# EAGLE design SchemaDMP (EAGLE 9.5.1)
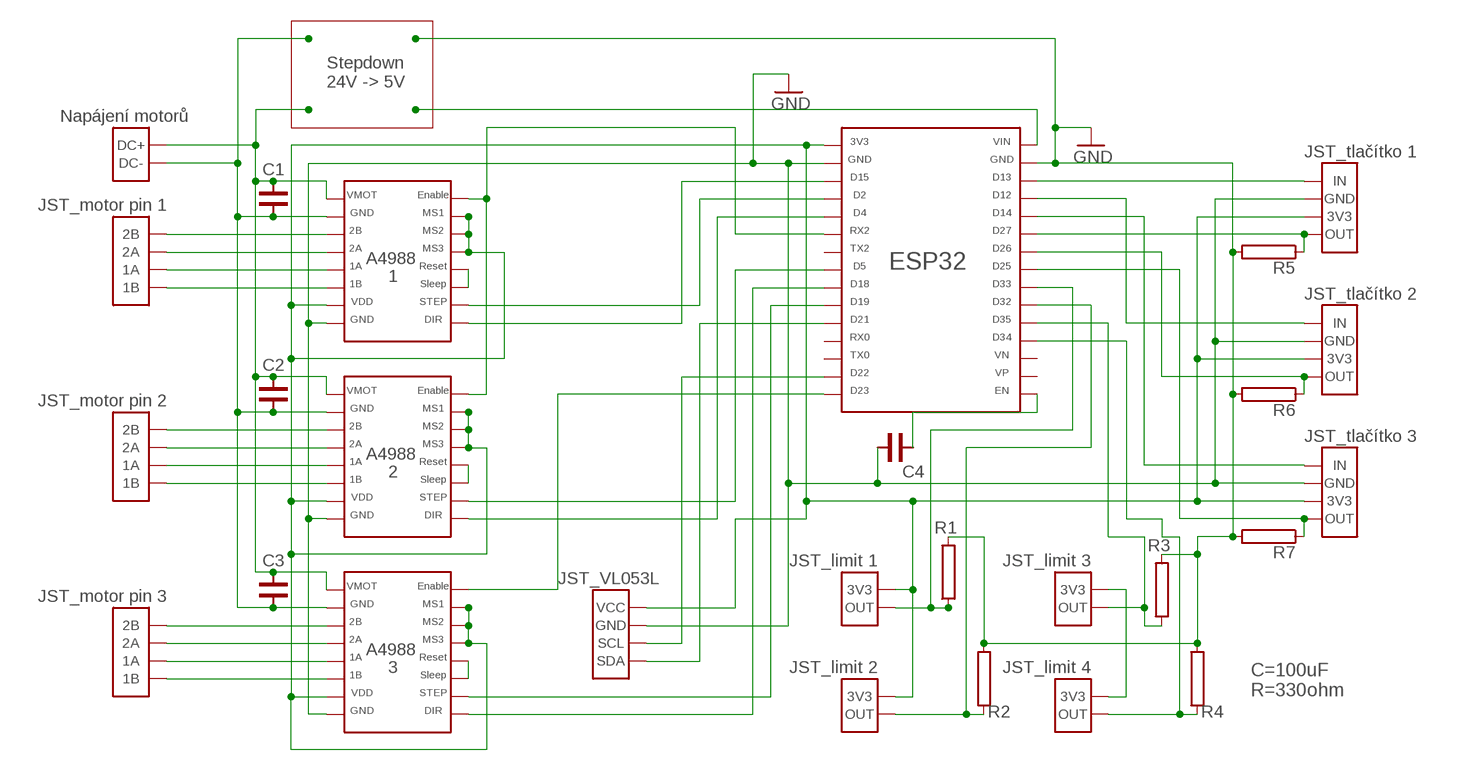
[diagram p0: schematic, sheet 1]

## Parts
R1  RR  [R]
R2  RR  [R]
R3  RR  [R]
R4  RR  [R]
R5  RR  [R]
R6  RR  [R]
R7  RR  [R]
U$1  A4988  [A4988]
U$2  A4988  [A4988]
U$3  JST_4P  [JST_4P]
U$4  JST_4P  [JST_4P]
U$5  A4988  [A4988]
U$6  JST_4P  [JST_4P]
U$7  POWER_2P  [POWER_2P]
U$8  ESP32  [ESP32]
U$9  JST_2P  [JST_2P]
U$10  JST_2P  [JST_2P]
U$11  JST_2P  [JST_2P]
U$12  JST_MOTOR  [JST_MOTOR]
U$13  JST_MOTOR  [JST_MOTOR]
U$14  JST_VL053L  [JST_VL053L]
U$15  JST_2P  [JST_2P]
U$16  JST_MOTOR  [JST_MOTOR]
U$18  C  [C]
U$19  C  [C]
U$20  C  [C]
U$22  STEPDOWN  [STEPDOWN]
U$23  C  [C]

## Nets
GND: R1.2 R2.2 R3.2 R4.2 R5.2 R6.2 R7.2 U$1.P$8(GND2) U$2.P$8(GND2) U$3.P$2 U$4.P$2 U$5.P$8(GND2) U$6.P$2 U$8.P$2(GND) U$8.P$17(GND2) U$14.P$2 U$22.P$1 U$23.P$1
N$2: U$1.P$2(GND) U$2.P$2(GND) U$5.P$2(GND) U$7.P$2 U$18.P$1 U$19.P$1 U$20.P$1 U$22.P$4
N$3: U$5.P$3(2B) U$12.P$1
N$4: U$5.P$4(2A) U$12.P$2
N$5: U$5.P$5(1A) U$12.P$3
N$6: U$5.P$6(1B) U$12.P$4
N$7: U$1.P$3(2B) U$13.P$1
N$8: U$1.P$4(2A) U$13.P$2
N$9: U$1.P$5(1A) U$13.P$3
N$10: U$1.P$6(1B) U$13.P$4
N$11: U$2.P$3(2B) U$16.P$1
N$12: U$2.P$4(2A) U$16.P$2
N$13: U$2.P$5(1A) U$16.P$3
N$14: U$2.P$6(1B) U$16.P$4
N$15: U$5.P$16(DIR) U$8.P$18(D15)
N$17: U$1.P$9(ENABLE) U$5.P$9(ENABLE) U$8.P$21(RX2)
N$19: U$1.P$7(VDD) U$1.P$10(MS1) U$1.P$11(MS2) U$1.P$12(MS3) U$2.P$7(VDD) U$2.P$10(MS1) U$2.P$11(MS2) U$2.P$12(MS3) U$3.P$3 U$4.P$3 U$5.P$7(VDD) U$5.P$10(MS1) U$5.P$11(MS2) U$5.P$12(MS3) U$6.P$3 U$8.P$16(3V3) U$10.P$1 U$14.P$1 U$15.P$1
N$21: U$5.P$13(RESET) U$5.P$14(SLEEP)
N$22: U$1.P$13(RESET) U$1.P$14(SLEEP)
N$23: U$2.P$13(RESET) U$2.P$14(SLEEP)
N$24: R5.1 U$4.P$4 U$8.P$6(D27)
N$25: U$5.P$15(STEP) U$8.P$19(D2)
N$26: U$1.P$16(DIR) U$8.P$20(D4)
N$27: U$1.P$15(STEP) U$8.P$23(D5)
N$28: U$2.P$15(STEP) U$8.P$25(D19)
N$29: U$2.P$16(DIR) U$8.P$24(D18)
N$30: U$8.P$1(VIN) U$22.P$2
N$31: R2.1 U$8.P$10(D32) U$10.P$2
N$32: R3.1 U$8.P$11(D35) U$9.P$2
N$33: R4.1 U$8.P$12(D34) U$11.P$2
N$34: U$8.P$26(D21) U$14.P$4
N$35: U$8.P$29(D22) U$14.P$3
N$36: U$4.P$1 U$8.P$3(D13)
N$37: U$6.P$1 U$8.P$4(D12)
N$38: U$3.P$1 U$8.P$5(D14)
N$39: R6.1 U$6.P$4 U$8.P$7(D26)
N$40: R7.1 U$3.P$4 U$8.P$8(D25)
N$41: U$2.P$9(ENABLE) U$8.P$30(D23)
N$44: U$8.P$15(EN) U$23.P$2
N$45: R1.1 U$8.P$9(D33) U$15.P$2
N$49: U$9.P$1 U$11.P$1
N$51: U$1.P$1(VMOT) U$2.P$1(VMOT) U$5.P$1(VMOT) U$7.P$1 U$18.P$2 U$19.P$2 U$20.P$2 U$22.P$3
Unconnected: U$8.P$13(VN) U$8.P$14(VP) U$8.P$22(TX2) U$8.P$27(RX0) U$8.P$28(TX0)

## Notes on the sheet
- Stepdown 
  24V -> 5V
- Napájení motorů
- JST_tlačítko 1
- C1
- JST_motor pin 1
- 1
- JST_tlačítko 2
- C2
- JST_motor pin 2
- JST_tlačítko 3
- 2 | C4
- C3 | JST_limit 1 | JST_limit 3
- JST_motor pin 3
- 3 | JST_limit 2 | JST_limit 4
- C=100uF
  R=330ohm

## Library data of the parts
R1-R7 = _DMP:R
U$1 U$2 U$5 = _DMP:A4988
U$3 U$4 U$6 = _DMP:JST_4P
U$7 = _DMP:POWER_2P
U$8 = _DMP:ESP32
U$9-U$11 U$15 = _DMP:JST_2P
U$12 U$13 U$16 = _DMP:JST_MOTOR
U$14 = _DMP:JST_VL053L
U$18-U$20 U$23 = _DMP:C
U$22 = _DMP:STEPDOWN

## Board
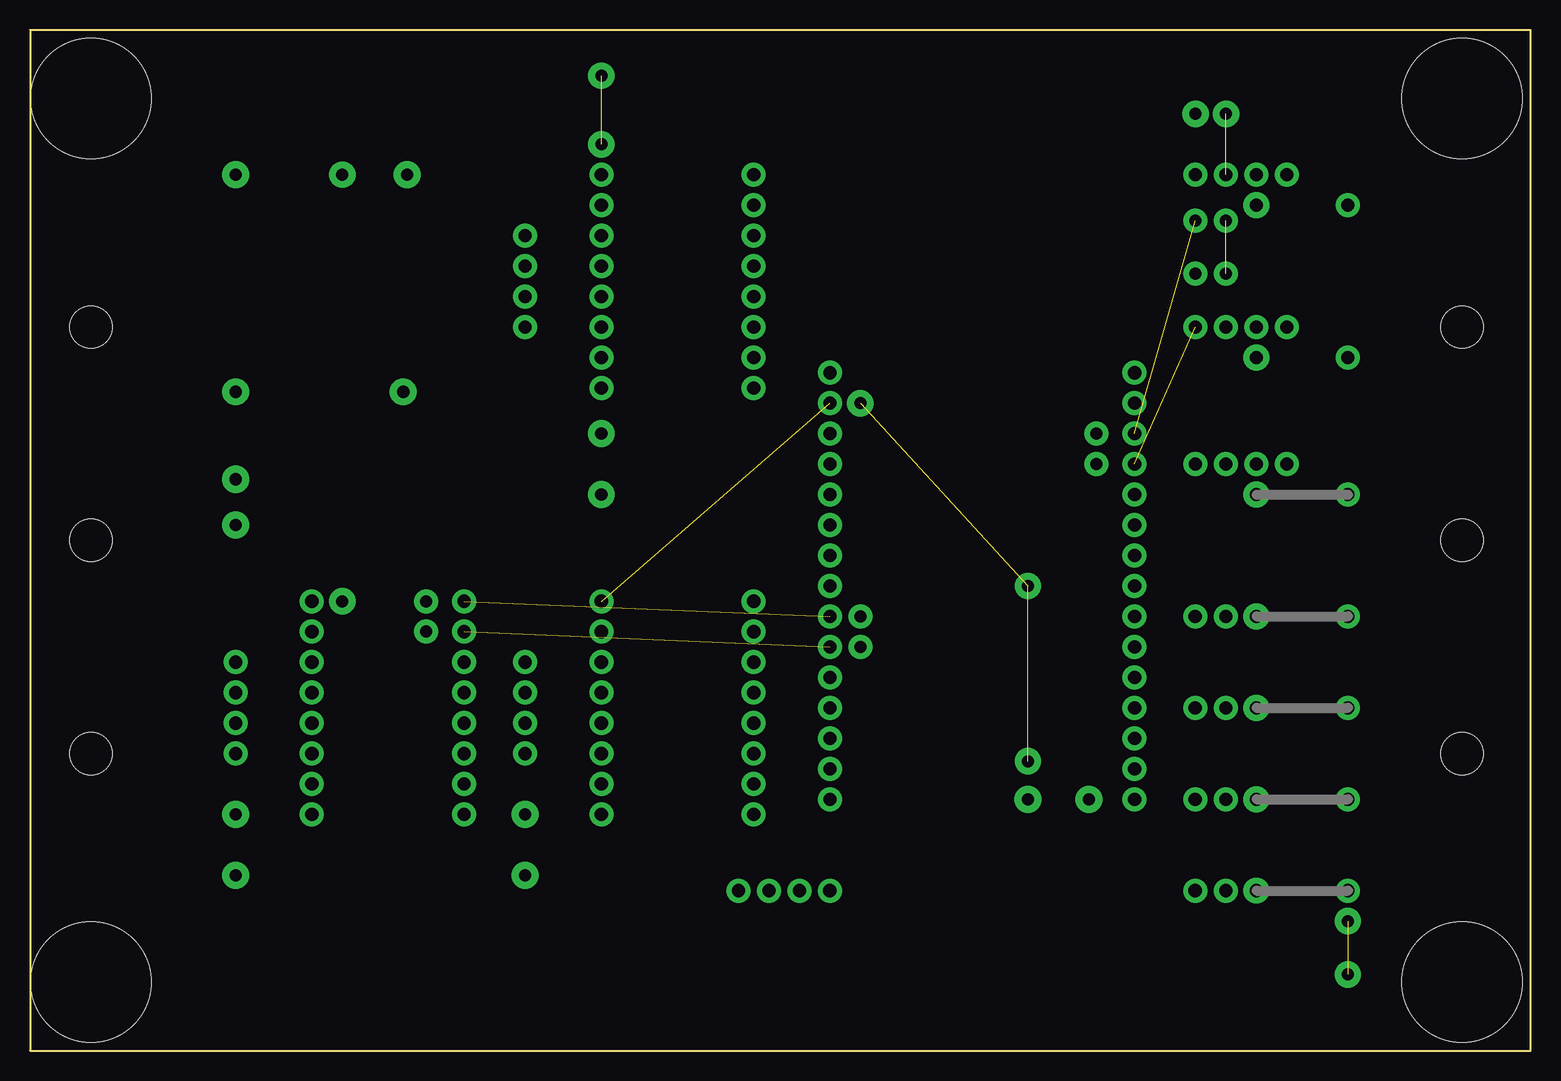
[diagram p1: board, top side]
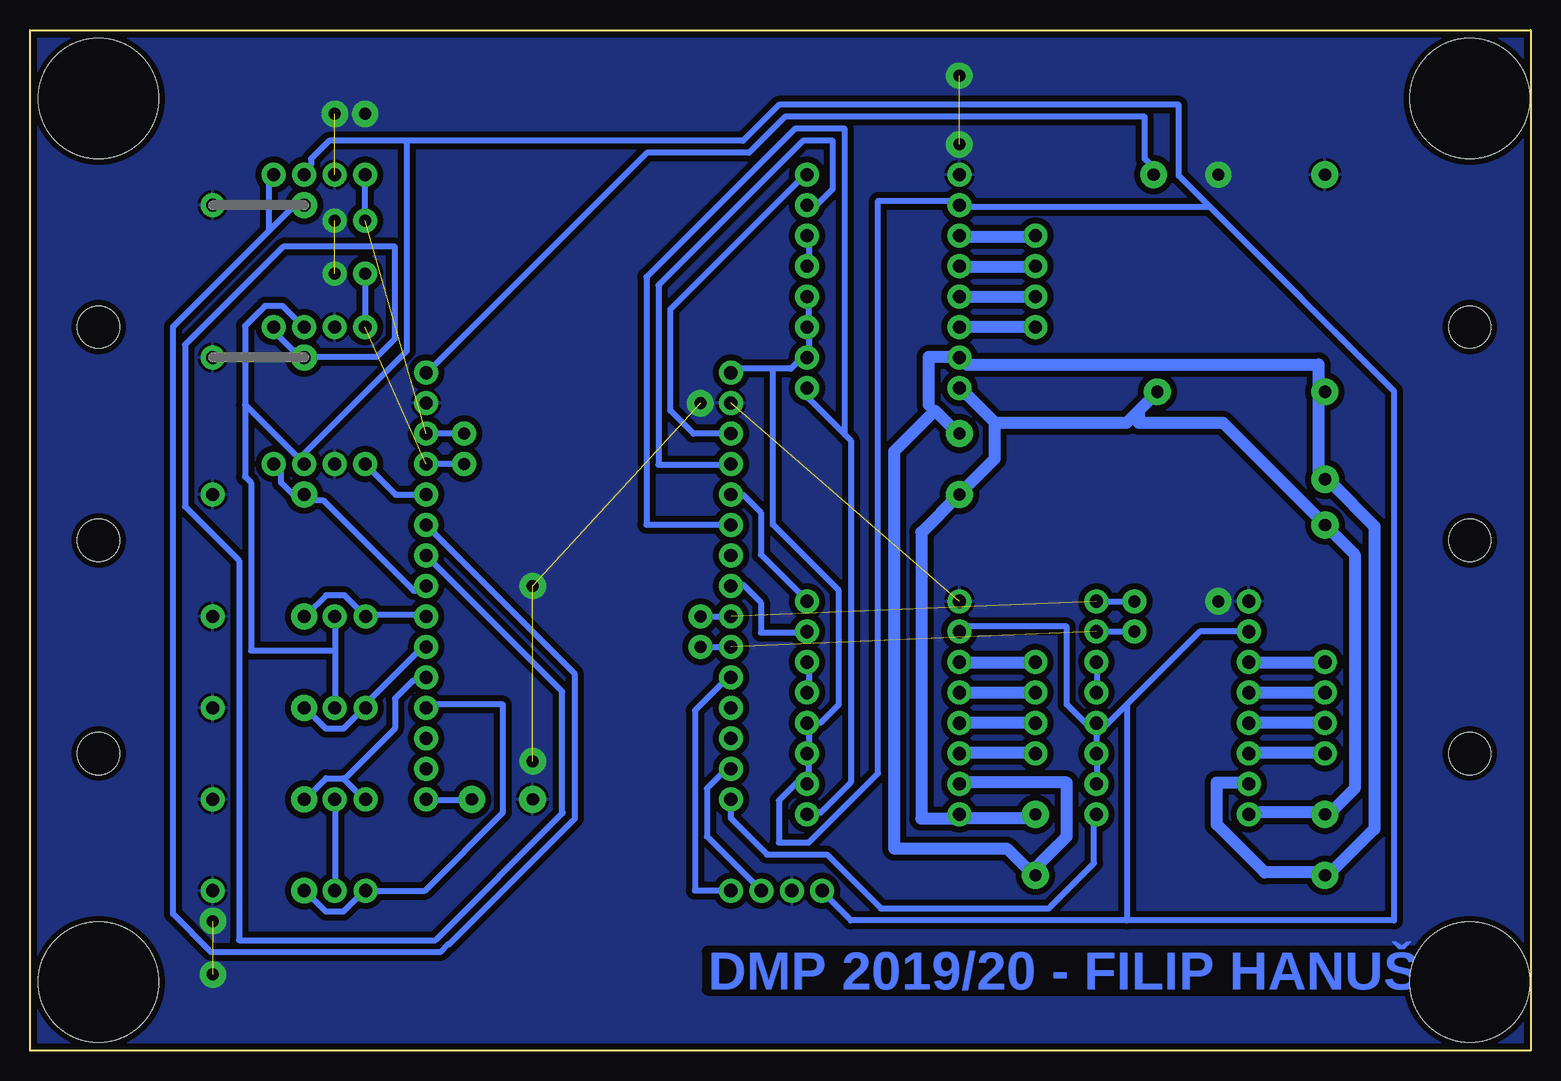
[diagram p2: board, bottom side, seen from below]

Size 125.09 x 85.09 mm. Coordinates in mm from the lower left corner, seen from the top.
Outline: 0,0 125.09,0 125.09,85.09 0,85.09 0,0
Copper layers (1*16): Top 0.035mm / dielectric 1.5mm / Bottom 0.035mm
Design rules "default *": minimum track width 0.5mm, minimum drill 1mm, track to track 0.5mm, track to pad 0.5mm, pad to pad 0.3mm, via to via 0.5mm, smd to smd 0.3mm, copper to edge 0.5mm, drill to drill 0.5mm, minimum pad ring 10mil, minimum via ring 8mil, stop-mask expansion 4mil, vias tented up to drill 0mil, thermal gap 10mil
Holes 3.5 mm at 5.08,42.55 119.38,42.55 5.08,60.33 5.08,24.77 119.38,60.33 119.38,24.77
Holes 10 mm at 5.08,79.38 119.38,79.38 119.38,5.71 5.08,5.71

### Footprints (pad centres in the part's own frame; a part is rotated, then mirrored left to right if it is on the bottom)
R = drill 1.1 pad 2.15: 1 0,0 | drill 1.1 pad 2: 2 7.62,0
A4988 = drill 1.1 pad 2: P$1 0,0; P$2 2.54,0; P$3 5.08,0; P$4 7.62,0; P$5 10.16,0; P$6 12.7,0; P$7 15.24,0; P$8 17.78,0; P$9 0,-12.7; P$10 2.54,-12.7; P$11 5.08,-12.7; P$12 7.62,-12.7; P$13 10.16,-12.7; P$14 12.7,-12.7; P$15 15.24,-12.7; P$16 17.78,-12.7
JST_4P = drill 1.1 pad 2: P$1 0,0; P$2 0,-2.54; P$3 0,-5.08; P$4 0,-7.62
POWER_2P = drill 1.02 pad 2.27: P$1 0,1.27; P$2 0,-2.54
ESP32 = drill 1.1 pad 2: P$1 0,0; P$2 2.54,0; P$3 5.08,0; P$4 7.62,0; P$5 10.16,0; P$6 12.7,0; P$7 15.24,0; P$8 17.78,0; P$9 20.32,0; P$10 22.86,0; P$11 25.4,0; P$12 27.94,0; P$13 30.48,0; P$14 33.02,0; P$15 35.56,0; P$16 0,-25.4; P$17 2.54,-25.4; P$18 5.08,-25.4; P$19 7.62,-25.4; P$20 10.16,-25.4; P$21 12.7,-25.4; P$22 15.24,-25.4; P$23 17.78,-25.4; P$24 20.32,-25.4; P$25 22.86,-25.4; P$26 25.4,-25.4; P$27 27.94,-25.4; P$28 30.48,-25.4; P$29 33.02,-25.4; P$30 35.56,-25.4
JST_2P = drill 1.1 pad 2: P$1 0,0; P$2 0,-2.57
JST_MOTOR = drill 1.1 pad 2: P$1 0,0; P$2 0,-2.54; P$3 0,-5.08; P$4 0,-7.62
JST_VL053L = drill 1.1 pad 2: P$1 0,0; P$2 0,-2.54; P$3 0,-5.08; P$4 0,-7.62
C = drill 1.02 pad 2.24: P$1 0,0; P$2 5.08,0
STEPDOWN = drill 1.02 pad 2.24: P$1 0,0; P$2 0,14.287; P$3 18.098,13.97; P$4 18.098,0

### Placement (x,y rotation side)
R1  102.23,36.2 0 top
R2  102.23,28.57 0 top
R3  102.23,20.95 0 top
R4  102.23,13.34 0 top
R5  102.23,70.48 180 bottom
R6  102.23,57.78 180 bottom
R7  102.23,46.35 0 top
U$1  47.62,19.68 90 top
U$2  23.5,19.68 90 top
U$3  97.16,48.9 90 top
U$4  97.16,73.03 90 top
U$5  47.62,55.24 90 top
U$6  97.16,60.33 90 top
U$7  17.14,45.09 180 top
U$8  92.08,56.52 270 top
U$9  99.69,20.95 270 top
U$10  99.69,28.57 270 top
U$11  99.69,13.34 270 top
U$12  41.27,60.33 180 top
U$13  41.27,24.77 180 top
U$14  59.05,13.34 90 top
U$15  99.69,36.2 270 top
U$16  17.14,24.77 180 top
U$18  17.14,14.61 90 top
U$19  41.27,14.61 90 top
U$20  47.62,51.44 270 top
U$22  17.14,73.03 270 top
U$23  83.19,20.95 0 top

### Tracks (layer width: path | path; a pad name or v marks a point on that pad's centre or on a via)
GND  (via drill 1 pad 2, 1 pad 2.2)  (7 unrouted)
  other vias: 47.62,75.56 47.62,81.28 69.22,53.98 99.69,78.11 109.86,6.35 83.19,24.13 83.19,38.73 99.69,69.22 99.69,64.77 97.16,78.11 109.86,10.79 26.04,37.47 26.04,73.03
  pour Bottom: 0,85.09 0,0 125.09,0 125.09,85.09
N$2
  Bottom 0.5: 41.16,15.35 41.16,14.85 U$19.P$1 41.66,14.85 | 47.16,22.35 U$1.P$2 | 23.66,22.35 U$2.P$2 | 17.16,14.85 U$18.P$1 16.66,14.85 | 49.66,53.35 50.16,53.85 | 47.66,57.85 U$5.P$2 | 47.66,51.35 U$20.P$1 | 17.66,48.35 17.16,47.85 U$7.P$2 16.66,47.35 | 17.66,54.35 17.16,54.85 U$22.P$4 17.66,54.35
  Bottom 1: 47.16,22.35 38.66,22.35 38.66,17.85 41.16,15.35 | 23.66,22.35 26.16,22.35 26.16,18.85 22.16,14.85 17.16,14.85 | 47.66,57.85 50.16,57.85 50.16,53.85 | 47.66,51.35 49.66,53.35 53.06,49.95 53.06,16.85 43.66,16.85 41.66,14.85 | 17.66,48.35 17.66,54.35 17.66,57.22 47.05,57.22 U$5.P$2 | 16.66,14.85 13.03,18.48 13.03,43.72 16.66,47.35
N$3
  Bottom 0.5: 41.66,60.35 U$12.P$1 | 47.16,60.35 U$5.P$3
  Bottom 1: 47.16,60.35 41.66,60.35
N$4
  Bottom 0.5: 41.66,62.85 U$12.P$2 | 47.16,62.85 U$5.P$4
  Bottom 1: 47.16,62.85 41.66,62.85
N$5
  Bottom 0.5: 41.66,65.35 U$12.P$3 | 47.16,65.35 U$5.P$5
  Bottom 1: 47.16,65.35 41.66,65.35
N$6
  Bottom 0.5: 41.66,67.85 U$12.P$4 | 47.16,67.85 U$5.P$6
  Bottom 1: 47.16,67.85 41.66,67.85
N$7
  Bottom 0.5: 41.66,24.85 U$13.P$1 | 47.16,24.85 U$1.P$3
  Bottom 1: 47.16,24.85 41.66,24.85
N$8
  Bottom 0.5: 41.66,27.35 U$13.P$2 | 47.16,27.35 U$1.P$4
  Bottom 1: 47.16,27.35 41.66,27.35
N$9
  Bottom 0.5: 41.66,29.85 U$13.P$3 | 47.16,29.85 U$1.P$5
  Bottom 1: 47.16,29.85 41.66,29.85
N$10
  Bottom 0.5: 41.66,32.35 U$13.P$4 | 47.16,32.35 U$1.P$6
  Bottom 1: 47.16,32.35 41.66,32.35
N$11
  Bottom 0.5: 17.16,24.85 U$16.P$1 | 23.16,24.85 U$2.P$3
  Bottom 1: 23.16,24.85 17.16,24.85
N$12
  Bottom 0.5: 17.16,27.35 U$16.P$2 | 23.16,27.35 U$2.P$4
  Bottom 1: 23.16,27.35 17.16,27.35
N$13
  Bottom 0.5: 17.16,29.85 U$16.P$3 | 23.16,29.85 U$2.P$5
  Bottom 1: 23.16,29.85 17.16,29.85
N$14
  Bottom 0.5: 17.16,32.35 U$16.P$4 | 23.16,32.35 U$2.P$6
  Bottom 1: 23.16,32.35 17.16,32.35
N$15
  Bottom 0.5: U$5.P$16 60.66,72.85 71.7,61.81 71.7,53.35 69.78,51.44 U$8.P$18
N$17
  Bottom 0.5: 57.16,51.35 60.16,54.35 60.16,54.85 U$5.P$9 | 57.16,51.35 56.66,50.85 56.66,22.35 59.16,19.85 60.16,19.85 U$1.P$9 | 57.16,51.35 57.16,76.85 61.34,76.85 73.7,64.49 73.7,43.85 67.16,43.85 U$8.P$21
N$19
  Bottom 0.5: U$2.P$10 36.16,22.35 36.16,24.35 U$2.P$11 36.16,24.85 36.16,26.35 | 36.16,26.35 36.16,26.85 U$2.P$12 | 36.16,26.35 33.66,28.85 | 23.66,34.85 U$2.P$7 27.59,34.92 33.66,28.85 | 36.16,26.35 U$2.P$12 | U$1.P$7 47.16,35.35 38.66,35.35 38.66,28.85 36.66,26.85 U$2.P$12 | 33.66,10.85 56.66,10.85 58.66,12.85 U$14.P$1 | 33.66,28.85 33.66,10.85 | 99.66,33.35 99.66,35.85 U$15.P$1 | 99.66,33.35 99.66,28.85 U$10.P$1 | 107.16,53.85 102.66,49.35 U$3.P$3 102.16,49.35 102.16,49.85 93.66,58.35 93.66,75.85 | 102.66,60.35 U$6.P$3 102.3,60.33 104.05,62.08 105.5,62.08 107.16,60.41 107.16,53.85 | 93.66,75.85 100.16,75.85 101.66,74.35 101.66,73.85 102.16,73.35 U$4.P$3 | 99.66,33.35 106.66,33.35 106.66,47.35 107.16,47.85 107.16,53.85 | 63.16,56.85 61.66,56.85 60.66,57.85 U$5.P$10 60.16,57.85 60.16,59.85 U$5.P$11 60.16,60.35 60.16,62.85 U$5.P$12 | 63.16,56.85 66.66,56.85 U$8.P$16 | 60.16,22.85 60.66,22.85 62.66,20.85 62.66,17.35 60.16,17.35 54.39,23.12 54.39,70.85 47.66,70.85 U$5.P$7 47.16,70.35 26.85,70.35 26.8,70.4 | 60.16,22.85 60.16,22.35 U$1.P$10 60.16,22.85 | 60.16,22.85 60.16,24.35 U$1.P$11 60.16,24.85 60.16,26.85 U$1.P$12 60.16,27.35 59.16,27.35 57.66,28.85 57.66,38.35 63.16,43.85 63.16,56.85 | 93.66,75.85 65.66,75.85 62.66,78.85 29.34,78.85 29.34,72.94 26.8,70.4 | 33.66,10.85 11.39,10.85 11.39,54.98 26.8,70.4
N$21
  Bottom 0.5: U$5.P$13 60.16,65.85 60.16,67.85 U$5.P$14
N$22
  Bottom 0.5: U$1.P$13 60.16,29.85 60.16,32.35 U$1.P$14
N$23
  Bottom 0.5: U$2.P$13 36.16,29.85 36.16,32.35 U$2.P$14
N$24
  Bottom 0.5: 90.16,8.85 90.14,8.87 | 90.14,8.87 79.66,19.35 79.66,31.4 U$8.P$6 91.66,43.85 | 105.16,68.35 102.66,70.85 R5.1 | 105.16,68.35 113.16,60.35 113.16,11.4 109.98,8.21 90.88,8.21 90.23,8.87 90.14,8.87 | 105.16,68.35 105.16,72.85 U$4.P$4
N$25
  Bottom 0.5: U$8.P$19 67.16,48.85 72.7,48.85 72.7,63.81 60.66,75.85 58.16,75.85 58.16,71.85 59.66,70.35 60.16,70.35 U$5.P$15
N$26
  Bottom 0.5: U$1.P$16 60.66,37.85 64.16,41.35 64.16,44.85 65.66,46.35 66.66,46.35 U$8.P$20
N$27
  Bottom 0.5: U$1.P$15 60.66,34.85 64.16,34.85 64.16,37.35 65.66,38.85 66.66,38.85 U$8.P$23
N$28  (via drill 1 pad 2)  (1 unrouted)
  Bottom 0.5: v69.22,33.66 U$8.P$25 | U$2.P$15 v33.02,34.92
N$29  (via drill 1 pad 2)  (1 unrouted)
  Bottom 0.5: v69.22,36.2 U$8.P$24 | U$2.P$16 v33.02,37.47
N$30
  Bottom 0.5: U$8.P$1 91.66,56.85 73.66,74.85 65.16,74.85 62.16,77.85 32.16,77.85 32.16,74.35 31.66,73.85 31.66,73.35 U$22.P$2
N$31
  Bottom 0.5: U$10.P$2 97.12,28.89 92.16,33.85 U$8.P$10 | 102.16,28.35 R2.1 102.17,28.57 100.42,26.82 98.97,26.82 97.22,28.57 U$10.P$2 | 97.16,28.35 U$10.P$2
N$32
  Bottom 0.5: 97.16,21.35 U$9.P$2 97.22,20.95 98.97,22.7 | 102.16,21.35 R3.1 102.17,20.95 100.42,22.7 98.97,22.7 | U$8.P$11 92.16,30.85 93.16,30.85 94.66,29.35 94.66,26.85 98.81,22.7 98.97,22.7
N$33
  Bottom 0.5: 97.16,12.85 U$11.P$2 | 102.16,12.85 R4.1 102.17,13.34 100.42,11.59 98.97,11.59 97.22,13.34 U$11.P$2 | U$8.P$12 91.66,28.85 85.66,28.85 85.66,19.85 92.17,13.34 U$11.P$2
N$34
  Bottom 0.5: U$14.P$4 67.16,13.35 69.66,13.35 69.66,28.35 67.16,30.85 U$8.P$26
N$35
  Bottom 0.5: U$14.P$3 64.16,13.35 68.66,17.85 68.66,21.85 67.16,23.35 U$8.P$29
N$36  (via drill 1 pad 2)  (1 unrouted)
  Bottom 0.5: v88.9,51.44 U$8.P$3 | v97.16,69.22 U$4.P$1
N$37  (via drill 1 pad 2)  (1 unrouted)
  Bottom 0.5: v88.9,48.9 U$8.P$4 | v97.16,64.77 U$6.P$1
N$38
  Bottom 0.5: U$3.P$1 94.62,46.36 94.62,46.35 92.16,46.35 U$8.P$5
N$39
  Bottom 0.5: 80.73,19.77 91.3,9.21 107.66,9.21 107.66,40.85 112.16,45.35 112.16,58.85 103.98,67.03 94.66,67.03 94.66,59.35 96.16,57.85 102.16,57.85 R6.1 102.66,57.85 102.66,58.35 103.16,58.35 104.66,59.85 U$6.P$4 | 80.73,19.77 80.66,19.85 | 91.66,41.35 U$8.P$7 80.73,29.93 80.73,19.77
N$40
  Bottom 0.5: 101.66,45.85 102.16,46.35 R7.1 101.66,45.85 | U$8.P$8 92.16,38.35 93.12,38.35 100.62,45.85 101.66,45.85 | 101.66,45.85 102.66,45.85 104.16,47.35 104.16,48.35 104.66,48.85 U$3.P$4
N$41
  Bottom 0.5: U$2.P$9 36.39,19.55 36.39,15.62 40.16,11.85 54.16,11.85 58.66,16.35 63.66,16.35 66.67,19.36 U$8.P$30
N$44
  Bottom 0.5: U$8.P$15 91.66,20.85 88.66,20.85 U$23.P$2
N$45
  Bottom 0.5: U$8.P$9 92.16,36.35 96.66,36.35 U$15.P$2 98.88,37.95 100.42,37.95 102.02,36.35 102.16,36.35 R1.1
N$49
  Bottom 0.5: U$11.P$1 99.66,13.35 99.66,20.85 U$9.P$1
N$51
  Bottom 0.5: 47.16,19.35 U$1.P$1 47.66,19.35 | 41.66,19.35 U$19.P$2 | 23.16,19.85 U$2.P$1 | 17.16,19.85 U$18.P$2 16.66,19.85 | 47.16,54.85 U$5.P$1 | 47.16,46.85 U$20.P$2 47.66,46.35 | 31.16,54.85 U$22.P$3 | 17.16,43.85 U$7.P$1 16.66,43.35
  Bottom 1: 41.66,19.35 47.16,19.35 | 17.16,19.85 23.16,19.85 | 44.66,52.35 47.16,54.85 | 44.66,52.35 44.66,49.35 47.16,46.85 | 32.66,53.35 33.66,52.35 44.66,52.35 | 32.66,53.35 31.16,54.85 | 17.16,43.85 25.66,52.35 32.66,52.35 32.66,53.35 | 16.66,19.85 14.66,21.85 14.66,41.35 16.66,43.35 | 47.66,19.35 50.8,19.35 50.8,43.22 47.66,46.35

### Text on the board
Bottom: DMP 2019/20 - FILIP HANUŠ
